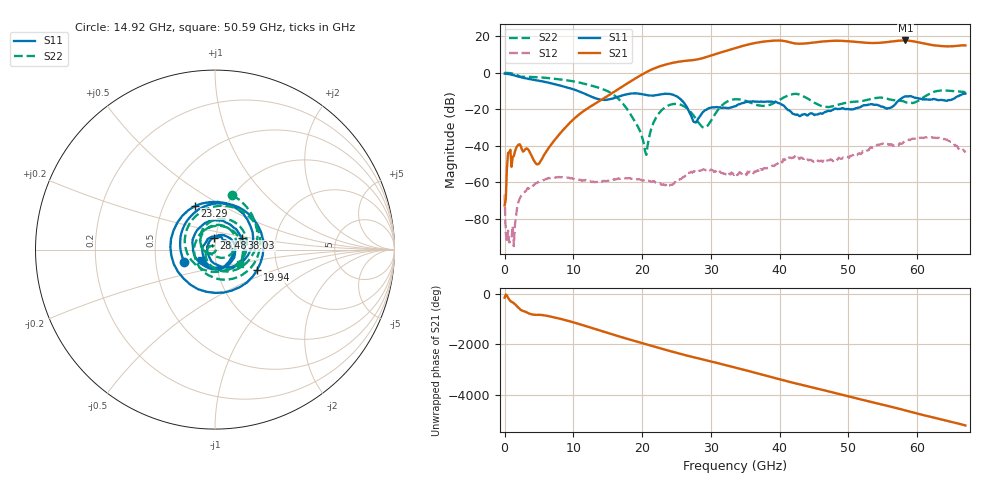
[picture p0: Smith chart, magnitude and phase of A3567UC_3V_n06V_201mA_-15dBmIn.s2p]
! MARKI MICROWAVE INC.
! Date:  4/20/2021
! Model Number:  A-3567UC
! Description:  2-port Small Signal S-parameter data for A-3567UC
! Frequency Range:  10 MHz to 67 GHz
! Port Configuration:  PORT 1: Input
!  PORT 2: Output
! Bias Condition: Vd = +3V, Vg = -0.6V, Id = 201mA
! A-3567UC s2p files are only valid for small signal conditions (below -10 dBm input power)
# Hz S  dB  R 50
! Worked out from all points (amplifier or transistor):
!   401 points, 10 MHz to 67 GHz, reference 50 ohm
!   highest |S21| = 17.8 dB at 58.29 GHz (marker M1)
!   |S21| within 3 dB of that: 34.63 GHz to 63.26 GHz (28.63 GHz wide, 58.5 % of centre)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
!   unconditionally stable (mu >= 1): 192 MHz to end of sweep
!   at 11.06 GHz: K = 3561.93, MAG = -20.3 dB, |S12| = -58.6 dB
!   at 33.51 GHz: K = 56.42, MAG = 13.8 dB, |S12| = -55.1 dB
!   at 67 GHz: K = 11.53, MAG = 15.8 dB, |S12| = -43.7 dB
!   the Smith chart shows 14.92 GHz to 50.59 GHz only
!   S11 on the Smith chart (normalised r, x): 14.92 GHz: 0.70, -0.10; 19.94 GHz: 1.56, -0.37; 23.29 GHz: 0.72, +0.38; 28.48 GHz: 0.98, +0.13; 38.03 GHz: 1.34, +0.18; 50.59 GHz: 0.85, -0.10
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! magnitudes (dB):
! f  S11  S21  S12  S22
! 10 MHz  -0.4  -72.7  -66.7  0.0
! 679.9 MHz  -0.7  -43.6  -93.1  -0.1
! 1.852 GHz  -1.9  -40.2  -73.1  -1.1
! 4.867 GHz  -4.2  -50.1  -59.9  -2.4
! 11.23 GHz  -10.7  -21.7  -59.2  -5.6
! 14.92 GHz  -14.7  -12.9  -59.2  -9.9
! 19.94 GHz  -11.7  -1.0  -58.9  -34.4
! 20.61 GHz  -12.2  0.4  -58.9  -44.9
! 22.45 GHz  -12.0  3.5  -60.9  -22.1
! 23.29 GHz  -11.5  4.4  -61.6  -19.0
! 25.8 GHz  -15.2  6.4  -57.8  -17.7
! 27.64 GHz  -27.0  7.1  -54.0  -24.2
! 28.48 GHz  -23.4  7.8  -53.6  -28.6
! 33.51 GHz  -18.3  13.6  -55.1  -14.5
! 38.03 GHz  -15.7  17.3  -52.5  -18.1
! 42.05 GHz  -22.6  16.3  -46.6  -11.5
! 44.73 GHz  -22.2  16.6  -48.2  -15.6
! 50.59 GHz  -20.1  17.2  -45.1  -15.9
! 55.95 GHz  -19.3  17.1  -39.6  -14.5
! 58.29 GHz  -12.8  17.8  -37.3  -16.1
! 63.32 GHz  -14.9  14.8  -35.8  -9.7
! 67 GHz  -11.4  15.1  -43.7  -10.6
